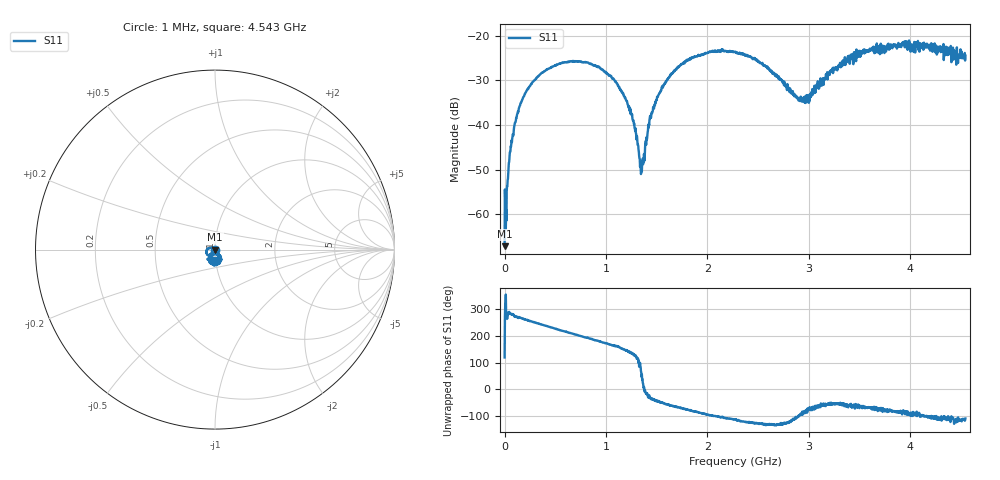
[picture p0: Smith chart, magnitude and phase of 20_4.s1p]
# HZ S RI R 50
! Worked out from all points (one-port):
!   1515 points, 1 MHz to 4.543 GHz, reference 50 ohm
!   lowest |S11| = -67.2 dB at 1 MHz (marker M1), VSWR 1.00, Z = 50 + j0.0382 ohm
!   |S11| at or under -10 dB: start of sweep to end of sweep
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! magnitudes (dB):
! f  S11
! 1 MHz  -67.2
! 25 MHz  -53.7
! 61 MHz  -44.8
! 112 MHz  -39.0
! 160 MHz  -35.1
! 226 MHz  -32.1
! 340 MHz  -28.9
! 571 MHz  -26.1
! 919 MHz  -27.0
! 1.138 GHz  -32.0
! 1.258 GHz  -37.6
! 1.3 GHz  -43.2
! 1.333 GHz  -47.6
! 1.357 GHz  -48.1
! 1.432 GHz  -38.4
! 1.486 GHz  -34.8
! 1.57 GHz  -31.1
! 1.705 GHz  -27.1
! 2.026 GHz  -23.6
! 2.272 GHz  -23.7
! 2.578 GHz  -27.0
! 2.842 GHz  -32.4
! 2.986 GHz  -33.3
! 3.214 GHz  -27.8
! 3.409 GHz  -25.1
! 3.616 GHz  -23.2
! 3.976 GHz  -21.7
! 4.543 GHz  -24.5
